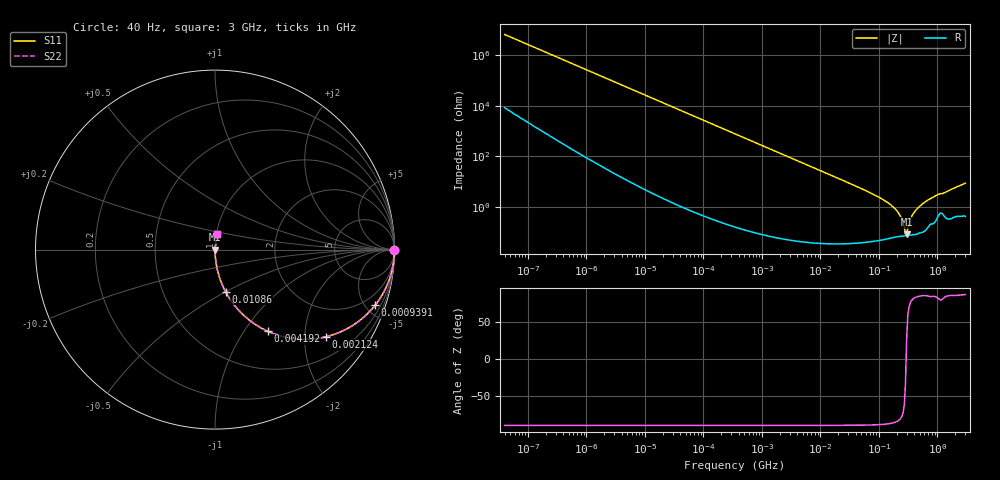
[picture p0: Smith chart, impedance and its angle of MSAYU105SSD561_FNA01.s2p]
! MSAYU105SSD561_FNA01  S-PARAMETER MODEL  ( General Type )
! Model Generated by TAIYO YUDEN Corporation (http://www.ty-top.com)
! Version 2.0
! TAIYO YUDEN Control No. 051115
! Copyright(c) 2005 TAIYO YUDEN CO.,LTD. All Rights Reserved.
! Product Description (link to TY-COMPAS)
! https://ds.yuden.co.jp/TYCOMPAS/or/detail?pn=MSAYU105SSD561KFNA01&u=M
! Products Name : Multilayer Ceramic Capacitors
! Characteristics :
!  Capacitance : 560 pF , Rated Voltage : 50V
!  Case Size : 1.0 x 0.5 / 0.039 x 0.02 [mm/inch] , Thickness : 0.5 / 0.02 [mm/inch]
!  (Conditions: Temperature = 25 degC , DC Bias Current/Voltage = 0A / 0V)
! External Node Assignments :
!  1  o---| |---o  2
! GND o---------o GND
! Frequency Range : 40Hz  -  3GHz  [ 401 STEP ]
# MHz S RI R 50
! Freq[MHz].  S11 Real  S11 Imag  S21 Real  S21 Imag  S12 Real  S12 Imag  S22 Real  S22 Imag
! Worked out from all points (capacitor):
!   401 points, 40 Hz to 3 GHz, reference 50 ohm
!   read as one part in series: C = 588 pF near 44 Hz
!   lowest |Z| = 80.2 mohm at 297.2 MHz (marker M1)
!   series resonance near 291.4 MHz, so ESL is about 510 pH
!   S11 on the Smith chart (normalised r, x): 40 Hz: open; 939.1 kHz: 1.00, -5.76; 2.124 MHz: 1.00, -2.55; 4.192 MHz: 1.00, -1.29; 10.86 MHz: 1.00, -0.50; 3 GHz: 1.01, +0.17
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4e-05  1 -1.48e-05  1.9e-08 1.48e-05  1.9e-08 1.48e-05  1 -1.48e-05
0.000257  1 -9.5e-05  6.1e-08 9.5e-05  6.1e-08 9.5e-05  1 -9.5e-05
0.000834  1 -0.000308  2.01e-07 0.000308  2.01e-07 0.000308  1 -0.000308
0.017386  1 -0.00643  4.23e-05 0.00643  4.23e-05 0.00643  1 -0.00643
0.362475  0.9823 -0.1316  0.0177 0.1316  0.0177 0.1316  0.9823 -0.1316
0.939115  0.8924 -0.3097  0.1076 0.3097  0.1076 0.3097  0.8924 -0.3097
2.123718  0.6187 -0.4855  0.3813 0.4855  0.3813 0.4855  0.6187 -0.4855
4.191906  0.2941 -0.4553  0.7059 0.4553  0.7059 0.4553  0.2941 -0.4553
7.222098  0.1232 -0.3282  0.8768 0.3282  0.8768 0.3282  0.1232 -0.3282
10.86056  0.0586 -0.2341  0.9414 0.2341  0.9414 0.2341  0.0586 -0.2341
63.63129  0.00203 -0.0404  0.998 0.0404  0.998 0.0404  0.00203 -0.0404
150.5692  0.000729 -0.0131  0.9993 0.0131  0.9993 0.0131  0.000729 -0.0131
216.3901  0.000695 -0.00557  0.9993 0.00557  0.9993 0.00557  0.000695 -0.00557
236.926  0.000693 -0.00383  0.9993 0.00383  0.9993 0.00383  0.000693 -0.00383
271.4411  0.000713 -0.00132  0.9993 0.00132  0.9993 0.00132  0.000713 -0.00132
297.2015  0.000715 0.000361  0.9993 -0.000361  0.9993 -0.000361  0.000715 0.000361
310.9844  0.000716 0.00121  0.9993 -0.00121  0.9993 -0.00121  0.000716 0.00121
356.2883  0.000772 0.00374  0.9992 -0.00374  0.9992 -0.00374  0.000772 0.00374
390.1008  0.000833 0.0055  0.9992 -0.0055  0.9992 -0.0055  0.000833 0.0055
560.6323  0.00114 0.0132  0.9989 -0.0132  0.9989 -0.0132  0.00114 0.0132
965.895  0.00396 0.0283  0.996 -0.0283  0.996 -0.0283  0.00396 0.0283
3000  0.0114 0.0847  0.9886 -0.0847  0.9886 -0.0847  0.0114 0.0847
